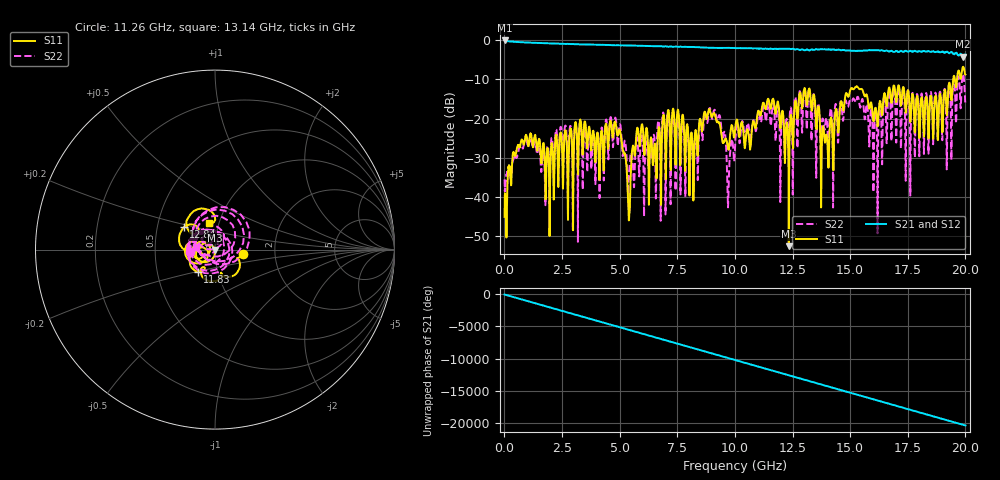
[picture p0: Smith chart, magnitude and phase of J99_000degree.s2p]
!Keysight Technologies,N5222A,MY51421036,A.10.65.16
!Date: Friday, March 31, 2023 15:04:05
!Correction: S11(Full 2 Port(1,2))
!S21(Full 2 Port(1,2))
!S12(Full 2 Port(1,2))
!S22(Full 2 Port(1,2))
!S2P File: Measurements: S11, S21, S12, S22:
# Hz S  dB  R 50
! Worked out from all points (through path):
!   2000 points, 10 MHz to 20 GHz, reference 50 ohm
!   highest |S21| = -0.02 dB at 10 MHz (marker M1); lowest = -4.1 dB at 19.9 GHz (marker M2)
!   group delay of S21, straight-line fit = 2.84 ns
!   lowest |S11| = -52.7 dB at 12.34 GHz (marker M3), VSWR 1.00, Z = 49.9 - j0.178 ohm
!   |S11| at or under -10 dB: start of sweep to 19.47 GHz; 19.54549 GHz to 19.63731 GHz (91.82 MHz wide, 0.469 % of centre)
!   |S22| runs from -51.6 to -8.6 dB; largest |S21 - S12| = 0.021
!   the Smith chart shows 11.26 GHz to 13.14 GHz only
!   S11 on the Smith chart (normalised r, x): 11.26 GHz: 1.37, -0.06; 11.83 GHz: 0.80, -0.20; 12.84 GHz: 0.68, +0.18; 13.14 GHz: 0.90, +0.28
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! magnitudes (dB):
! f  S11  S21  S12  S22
! 10 MHz  -45.1  0.0  -0.1  -35.6
! 680 MHz  -27.2  -0.5  -0.4  -27.3
! 1.88 GHz  -27.8  -0.8  -0.7  -27.2
! 3.35 GHz  -23.3  -1.0  -1.0  -24.4
! 4.88 GHz  -23.6  -1.3  -1.2  -23.4
! 5.39 GHz  -44.0  -1.3  -1.3  -36.2
! 5.82 GHz  -24.0  -1.4  -1.4  -30.5
! 6.68 GHz  -22.9  -1.5  -1.5  -20.5
! 10.01 GHz  -22.7  -2.0  -1.9  -27.1
! 11.26 GHz  -16.1  -2.2  -2.1  -17.2
! 11.83 GHz  -16.2  -2.2  -2.2  -18.0
! 12.34 GHz  -52.7  -2.1  -2.1  -26.0
! 12.84 GHz  -13.4  -2.4  -2.4  -13.5
! 13.14 GHz  -16.3  -2.3  -2.3  -19.4
! 13.34 GHz  -17.9  -2.3  -2.3  -22.5
! 13.99 GHz  -24.5  -2.3  -2.3  -20.3
! 15.09 GHz  -12.3  -2.7  -2.7  -15.5
! 16.1 GHz  -17.3  -2.5  -2.5  -18.1
! 16.67 GHz  -12.5  -2.8  -2.8  -13.1
! 18.71 GHz  -14.2  -3.0  -2.8  -13.5
! 19.9 GHz  -6.8  -4.1  -3.9  -8.6
! 20 GHz  -8.8  -3.6  -3.4  -15.9
